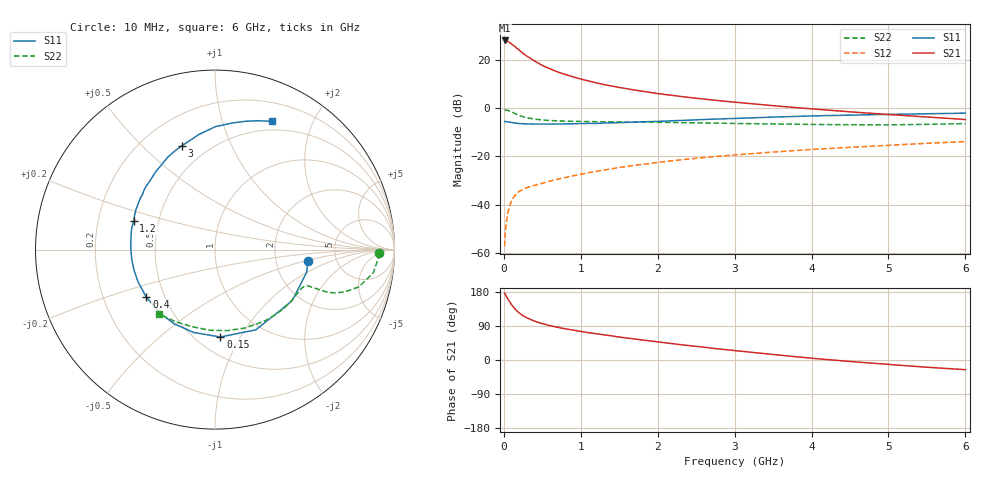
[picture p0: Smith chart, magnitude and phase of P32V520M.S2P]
! SIEMENS Small Signal Semiconductors
! BFP181
! Si NPN RF Bipolar Junction Transistor in SOT143
! VCE = 2.5 V  IC = 20 mA
! Common Emitter S-Parameters:  March  1996
# GHz  S  MA  R  50
!  f  S11  S21  S12  S22
! GHz  MAG  ANG  MAG  ANG  MAG  ANG  MAG  ANG
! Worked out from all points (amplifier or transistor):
!   36 points, 10 MHz to 6 GHz, reference 50 ohm
!   highest |S21| = 27.9 dB at 10 MHz (marker M1)
!   |S21| within 3 dB of that: start of sweep to 161.7 MHz
!   unconditionally stable (mu >= 1): start of sweep to 17.82 MHz; 400.3 MHz to end of sweep
!   at 250 MHz: K = 0.74, MSG = 28.1 dB, |S12| = -33.6 dB
!   at 1.4 GHz: K = 1.58, MAG = 12.6 dB, |S12| = -25.1 dB
!   at 6 GHz: K = 1.20, MAG = 1.9 dB, |S12| = -13.9 dB
!   S11 on the Smith chart (normalised r, x): 10 MHz: 3.07, -0.55; 150 MHz: 0.65, -0.83; 400 MHz: 0.40, -0.27; 1.2 GHz: 0.36, +0.15; 3 GHz: 0.36, +0.66; 6 GHz: 0.40, +1.46
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0.01  0.521 -7.2  24.75 176.2  0.0014 71.8  0.9161 -1.3
0.02  0.5261 -13.8  24.7 172.7  0.0029 81.8  0.9105 -3.1
0.05  0.5161 -33.5  23.82 161.7  0.0068 78.5  0.892 -8.3
0.1  0.5016 -63.0  21 145.9  0.0124 65.1  0.8285 -14.5
0.15  0.4879 -86.5  18.16 133.5  0.016 57.1  0.758 -18.2
0.2  0.4767 -104.5  15.6 124.1  0.019 54.1  0.7025 -20.1
0.25  0.4719 -118.5  13.39 116.7  0.0208 51.7  0.6597 -20.8
0.3  0.4678 -129.4  11.72 111.3  0.0227 50.1  0.6284 -21.0
0.4  0.4657 -145.2  9.289 102.4  0.0253 50.6  0.5882 -21.1
0.5  0.465 -157.1  7.565 96.0  0.0279 50.7  0.5644 -21.2
0.6  0.4653 -166.1  6.437 90.7  0.0309 52.5  0.5501 -21.5
0.7  0.4671 -173.1  5.521 86.3  0.0339 53.4  0.5411 -22.1
0.9  0.4711 175.4  4.388 79.0  0.0397 55.6  0.5297 -23.9
1.1  0.48 165.0  3.61 72.1  0.0461 56.1  0.5229 -26.1
1.2  0.4794 160.7  3.302 69.4  0.0489 56.6  0.5208 -27.5
1.7  0.5087 142.2  2.345 55.5  0.0656 56.2  0.511 -34.9
2.2  0.5447 127.6  1.808 42.9  0.0817 54.2  0.4998 -43.3
3  0.6068 107.8  1.316 24.9  0.1071 49.2  0.4782 -58.5
3.5  0.6479 97.9  1.114 14.5  0.1228 45.6  0.4674 -69.3
4.5  0.7106 82.6  0.832 -3.9  0.1538 37.4  0.4505 -93.8
5.5  0.7585 71.2  0.651 -19.1  0.1865 29.4  0.4584 -119.0
6  0.7807 66.2  0.577 -25.5  0.2017 24.8  0.4745 -131.2
